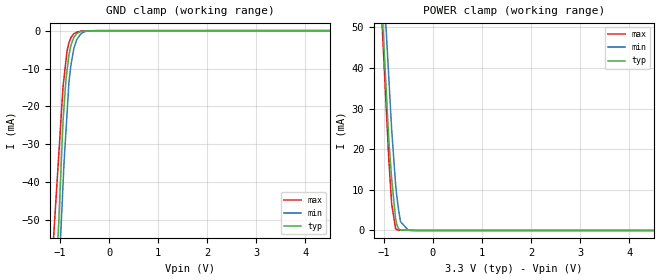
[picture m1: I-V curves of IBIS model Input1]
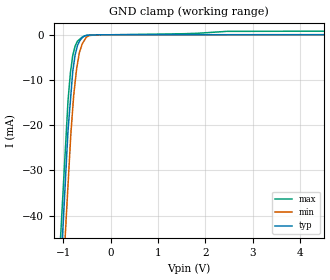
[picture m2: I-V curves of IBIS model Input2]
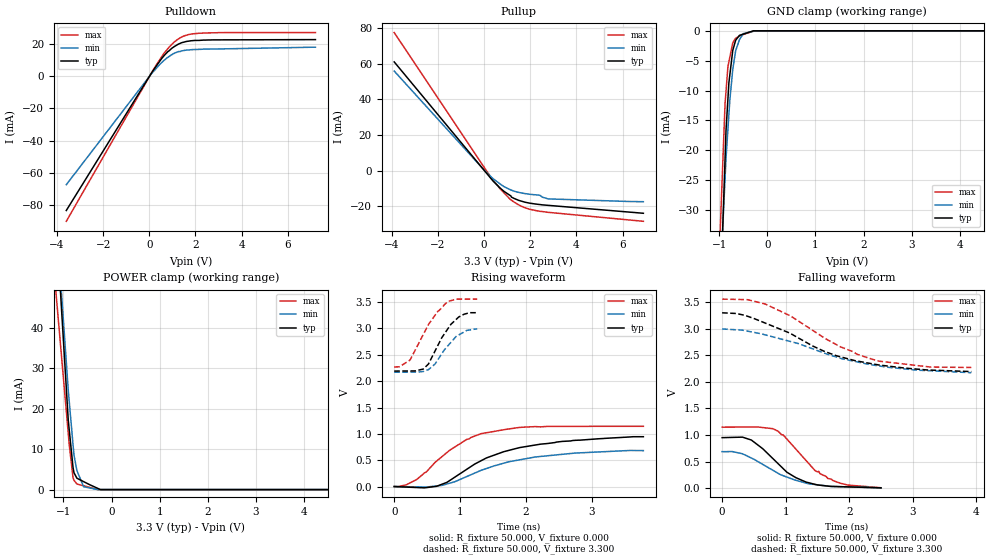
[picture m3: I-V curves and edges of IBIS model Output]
[IBIS Ver]   3.2
[Comment Char] |_char
[File Name]   ads1602ipfbt.ibs
[File Rev]   3.0
[Source]
| This model file was created by Teraspeed Consulting Group LLC
| (http://www.teraspeed.com/).
[Date]   08-30-2006
[Notes]   Quality Check of this IBIS model: Model Passes IBIS Check
   Model parses into ICX IS. Simulation done with Hyperlynx.
   1. MIN TYP MAX information is based on Temprature and Voltage
   characteristics only.
[Disclaimer]
| This model is designed as an aid for customers of Texas Instruments.
| TI and its licensors and suppliers make no warranties, either expressed
| or implied, with respect to this  model, including the warranties of
| merchantability or fitness for a particular purpose.
| The model is provided solely on an "as is" basis. The entire risk as to
| its quality and performance is with the customer.
[Copyright]
| (C) Copyright 2008 Texas Instruments Incorporated. All rights reserved.
[Component] ADS1602IPFBT
[Manufacturer] TI
[Package]
| variable   typ   min   max
R_pkg  1.8006E-02  1.8006E-02  1.8006E-02
L_pkg  2.1607E-09  2.1607E-09  2.1607E-09
C_pkg  6.0021E-13  6.0021E-13  6.0021E-13
[Pin] signal_name  model_name  R_pin  L_pin C_pin
1   AGND   GND   1.89E-02   2.26E-09   6.29E-13
2   AVDD   POWER   1.80E-02   2.16E-09   6.01E-13
3   AGND   GND   1.72E-02   2.06E-09   5.73E-13
4   AINN   Term1   1.64E-02   1.97E-09   5.47E-13
5   AINP   Term1   1.56E-02   1.87E-09   5.21E-13
6   AGND   GND   1.49E-02   1.78E-09   4.96E-13
7   AVDD   POWER   1.49E-02   1.78E-09   4.96E-13
8   RBIAS   Term1   1.56E-02   1.87E-09   5.21E-13
9   AGND   GND   1.64E-02   1.97E-09   5.47E-13
10   AVDD   POWER   1.72E-02   2.06E-09   5.73E-13
11   AGND   GND   1.80E-02   2.16E-09   6.01E-13
12   AVDD   POWER   1.89E-02   2.26E-09   6.29E-13
13   _REFEN  Input2  1.89E-02   2.26E-09   6.29E-13
14   NC   NC   1.80E-02   2.16E-09   6.01E-13
15   RPULLUP Term1   1.72E-02   2.06E-09   5.73E-13
16   NC   NC   1.64E-02   1.97E-09   5.47E-13
17   _PD   Input2  1.56E-02   1.87E-09   5.21E-13
18   DVDD   POWER   1.49E-02   1.78E-09   4.96E-13
19   DGND   GND   1.49E-02   1.78E-09   4.96E-13
20   SYNC   Input2  1.56E-02   1.87E-09   5.21E-13
21   OTR   Output  1.64E-02   1.97E-09   5.47E-13
22   DGND   GND   1.72E-02   2.06E-09   5.73E-13
23   DVDD   POWER   1.80E-02   2.16E-09   6.01E-13
24   NC   NC   1.89E-02   2.26E-09   6.29E-13
25   NC   NC   1.89E-02   2.26E-09   6.29E-13
26   NC   NC   1.80E-02   2.16E-09   6.01E-13
27   _SCLK   Output  1.72E-02   2.06E-09   5.73E-13
28   SCLK   Output  1.64E-02   1.97E-09   5.47E-13
29   _DOUT   Output  1.56E-02   1.87E-09   5.21E-13
30   DOUT   Output  1.49E-02   1.78E-09   4.96E-13
31   _FSO   Output  1.49E-02   1.78E-09   4.96E-13
32   FSO   Output  1.56E-02   1.87E-09   5.21E-13
33   DGND   GND   1.64E-02   1.97E-09   5.47E-13
34   DVDD   POWER   1.72E-02   2.06E-09   5.73E-13
35   NC   NC   1.80E-02   2.16E-09   6.01E-13
36   DGND   GND   1.89E-02   2.26E-09   6.29E-13
37   IOVDD   POWER   1.89E-02   2.26E-09   6.29E-13
38   DGND   GND   1.80E-02   2.16E-09   6.01E-13
39   AGND   GND   1.72E-02   2.06E-09   5.73E-13
40   CLK   Input1  1.64E-02   1.97E-09   5.47E-13
41   AGND   GND   1.56E-02   1.87E-09   5.21E-13
42   AVDD   POWER   1.49E-02   1.78E-09   4.96E-13
43   VCAP   Term1   1.49E-02   1.78E-09   4.96E-13
44   VREFN   Term1   1.56E-02   1.87E-09   5.21E-13
45   VREFN   Term1   1.64E-02   1.97E-09   5.47E-13
46   VMID   Term1   1.72E-02   2.06E-09   5.73E-13
47   VREFP   Term1   1.80E-02   2.16E-09   6.01E-13
48   VREFP   Term1   1.89E-02   2.26E-09   6.29E-13
[Diff Pin] inv_pin vdiff tdelay_typ tdelay_min tdelay_max
5   4   NA  NA  NA  NA
28  27  NA  NA  NA  NA
30  29  NA  NA  NA  NA
32  31  NA  NA  NA  NA
| Models and submodels in the file (4): Input1 (Input), Input2 (Input), Output (Output), Term1 (Terminator)
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[Model] Input1
Model_type Input
Vinl = 990.000mV
Vinh = 2.31000V
C_comp 2.00000pF 2.00000pF 2.00000pF
| variable typ   min   max
[Voltage Range] 3.30000V 3.00000V 3.60000V
[POWER Clamp Reference] 3.30000V 3.00000V 3.60000V
[GND Clamp Reference] 0.00000V 0.00000V 0.00000V
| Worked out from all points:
|   GND clamp passes 1 mA (typ) near -0.67 V on its own axis
|   POWER clamp passes 1 mA (typ) near -0.72 V on its own axis
[GND Clamp]
-3.3V     -742.8mA   -704.3mA   -501mA
-940mV    -23.81mA   -40.58mA   -14.84mA
-920mV    -20.15mA   -34.95mA   -12.5mA
-880mV    -12.82mA   -26.45mA   -7.834mA
-860mV    -10.7mA    -22.2mA    -5.498mA
-820mV    -6.461mA   -13.7mA    -3.17mA
-780mV    -3.9mA     -9.185mA   -1.829mA
-720mV    -1.771mA   -4.71mA    -825.5uA
-660mV    -787.2uA   -2.326mA   -383.3uA
-540mV    -168.5uA   -505.8uA   -71.65uA
-240mV    -9.723uA   -9.634uA   -1.75uA
6.6V      11.72uA    18.06uA    6.055uA
[POWER Clamp]
-3.3V     585.2mA    563.6mA    629.9mA
-1.06V    59.95mA    72.93mA    57.25mA
-1.02V    50.57mA    64.16mA    47.03mA
-900mV    22.43mA    37.88mA    17.72mA
-840mV    12.66mA    24.74mA    6.473mA
-760mV    2.906mA    11.27mA    428uA
-740mV    1.575mA    8.921mA    253.9uA
-700mV    404.3uA    5.099mA    76.65uA
-660mV    92.03uA    2.156mA    70.39uA
-500mV    47.41uA    57.43uA    45.36uA
6.6V      0A         0A         0A
[Model] Input2
Model_type Input
Vinl = 990.000mV
Vinh = 2.31000V
C_comp 2.00000pF 2.00000pF 2.00000pF
| variable typ   min   max
[Voltage Range] 3.30000V 3.00000V 3.60000V
[POWER Clamp Reference] 3.30000V 3.00000V 3.60000V
[GND Clamp Reference] 0.00000V 0.00000V 0.00000V
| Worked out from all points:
|   GND clamp passes 1 mA (typ) near -0.63 V on its own axis
[GND Clamp]
|  Voltage   I(typ)   I(min)   I(max)
-3.3V     -503.8mA   -490.3mA   -476.1mA
-900mV    -21.11mA   -33.25mA   -14.54mA
-840mV    -13.29mA   -21.82mA   -7.65mA
-800mV    -8.085mA   -16.2mA    -4.572mA
-780mV    -6.626mA   -13.39mA   -3.734mA
-750mV    -4.437mA   -10.5mA    -2.477mA
-720mV    -3.188mA   -7.613mA   -1.838mA
-660mV    -1.507mA   -3.925mA   -1.049mA
-550mV    -282.4uA   -1.149mA   -273.1uA
-440mV    -79.83uA   -142.4uA   -129uA
-220mV    -6.361uA   -5.894uA   -40uA
6.6V      14.04uA    12.24uA    839.7uA
[POWER Clamp]
-3.3V     0A         0A         0A
6.6V      0A         0A         0A
[Model] Output
Model_type Output
Vref=0.00000V
Rref=5.00000Mohms
Cref=0.00000F
Vmeas=1.65000V
C_comp 2.00000pF 2.00000pF 2.00000pF
| variable typ   min   max
[Voltage Range] 3.30000V 3.00000V 3.60000V
[POWER Clamp Reference] 3.30000V 3.00000V 3.60000V
[Pullup Reference] 3.30000V 3.00000V 3.60000V
[Pulldown Reference] 0.00000V 0.00000V 0.00000V
[GND Clamp Reference] 0.00000V 0.00000V 0.00000V
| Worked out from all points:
|   slope of the pulldown table from 0 to 0.495 V, typ, clamps not added: 47.7 ohm
|   slope of the pullup table from 0 to 0.495 V, typ, clamps not added: 66.9 ohm
|   GND clamp passes 1 mA (typ) near -0.60 V on its own axis
|   POWER clamp passes 1 mA (typ) near -0.41 V on its own axis
|   rising waveform, R_fixture 50.000, V_fixture 0.000: 20-80 % time 1.05ns typ, 1.07ns min, 714ps max; typ from 0.006 V to 0.95 V
|   falling waveform, R_fixture 50.000, V_fixture 0.000: 20-80 % time 548ps typ, 690ps min, 585ps max; typ from 0.95 V to 0.006 V
|   falling waveform, R_fixture 50.000, V_fixture 3.300: 20-80 % time 1.31ns typ, 1.43ns min, 1.14ns max; typ from 3.3 V to 2.19 V
|   rising waveform, R_fixture 50.000, V_fixture 3.300: 20-80 % time 304ps typ, 301ps min, 355ps max; typ from 2.19 V to 3.3 V
[GND Clamp]
-3.6V     -671.8mA   -487.7mA   -586.5mA
-3V       -528.4mA   -385.6mA   -459.8mA
-880mV    -21.47mA   -24.75mA   -12.22mA
-860mV    -16.69mA   -21.34mA   -10.14mA
-820mV    -11.37mA   -16.46mA   -5.974mA
-800mV    -8.704mA   -14.02mA   -5.185mA
-780mV    -7.354mA   -11.57mA   -4.396mA
-720mV    -3.302mA   -6.494mA   -2.028mA
-660mV    -1.589mA   -3.363mA   -1.234mA
-500mV    -548.3uA   -478.1uA   -619.2uA
-270mV    0A         -38.25uA   0A
7.2V      0A         0A         0A
[Pulldown]
-3.6V     -83.44mA   -67.43mA   -90.14mA
140mV     2.973mA    2.239mA    3.125mA
640mV     12.72mA    9.781mA    14.21mA
980mV     17.33mA    13.34mA    19.74mA
1.22V     19.5mA     15.01mA    22.68mA
1.44V     20.86mA    15.73mA    24.53mA
1.72V     21.72mA    16.18mA    25.83mA
2.36V     22.34mA    16.72mA    26.75mA
7.2V      22.63mA    17.95mA    27.01mA
[Pullup]
|  Voltage   I(typ)   I(min)   I(max)
-3.9V     60.97mA    55.83mA    77.43mA
0V        97.14uA    239.5uA    1.807mA
300mV     -4.585mA   -3.553mA   -3.954mA
720mV     -10.18mA   -7.819mA   -10.71mA
1.16V     -14.31mA   -10.92mA   -16.51mA
1.18V     -14.89mA   -11.01mA   -16.68mA
1.3V      -15.68mA   -11.59mA   -17.72mA
1.76V     -17.74mA   -12.93mA   -20.86mA
2.4V      -19.07mA   -13.83mA   -22.86mA
2.54V     -19.29mA   -15.03mA   -23.05mA
2.78V     -19.55mA   -15.93mA   -23.47mA
6.9V      -23.98mA   -17.49mA   -28.49mA
[POWER Clamp]
-3.9V     606.6mA    538.6mA    422.6mA
-1.14V    64.33mA    65.7mA     46.6mA
-1.06V    48.61mA    52mA       35.71mA
-970mV    30.93mA    36.58mA    23.44mA
-900mV    17.18mA    24.58mA    13.91mA
-880mV    14.82mA    21.87mA    11.18mA
-800mV    5.406mA    11.01mA    2.89mA
-780mV    4.158mA    8.472mA    2.298mA
-720mV    2.815mA    4.701mA    1.381mA
-580mV    1.97mA     710.8uA    976.2uA
-230mV    0A         0A         0A
6.9V      0A         0A         0A
[Rising Waveform]
R_fixture = 50.000
V_fixture = 0.000
V_fixture_min = 0.000
V_fixture_max = 0.000
|  time   V(typ)   V(min)   V(max)
0s        6.072mV    6.82mV     8.158mV
180ps     -3.481mV   3.037mV    36.74mV
340ps     -11.97mV   -326.8uV   138.7mV
640ps     10.32mV    16.91mV    484.3mV
800ps     85.89mV    55.34mV    650.4mV
1.1ns     332.4mV    195.3mV    898.3mV
1.32ns    496.3mV    314.4mV    1.008V
1.66ns    665.5mV    448mV      1.081V
2.22ns    809mV      575.9mV    1.136V
3.78ns    949.7mV    686.6mV    1.147V
[Falling Waveform]
R_fixture = 50.000
V_fixture = 0.000
V_fixture_min = 0.000
V_fixture_max = 0.000
|  time   V(typ)   V(min)   V(max)
0s        949.7mV    686.6mV    1.147V
320ps     959.7mV    647.1mV    1.149V
460ps     905mV      566.8mV    1.15V
800ps     555mV      335.9mV    1.118V
1.02ns    299mV      208.4mV    922.1mV
1.32ns    114.9mV    95.77mV    520.9mV
1.46ns    72.61mV    68.56mV    333.6mV
1.66ns    39.55mV    40.59mV    183.8mV
1.86ns    28.66mV    27.64mV    92.84mV
2.5ns     6.072mV    6.82mV     8.158mV
[Falling Waveform]
R_fixture = 50.000
V_fixture = 3.300
V_fixture_min = 3.000
V_fixture_max = 3.600
|  time   V(typ)   V(min)   V(max)
0s        3.297V     2.993V     3.554V
360ps     3.249V     2.961V     3.545V
680ps     3.103V     2.882V     3.461V
1.08ns    2.905V     2.756V     3.235V
1.6ns     2.576V     2.542V     2.83V
2.12ns    2.391V     2.375V     2.519V
2.36ns    2.339V     2.317V     2.424V
2.48ns    2.314V     2.296V     2.386V
3.28ns    2.22V      2.207V     2.277V
3.92ns    2.192V     2.171V     2.269V
[Rising Waveform]
R_fixture = 50.000
V_fixture = 3.300
V_fixture_min = 3.000
V_fixture_max = 3.600
|  time   V(typ)   V(min)   V(max)
0s        2.192V     2.171V     2.269V
80ps      2.193V     2.171V     2.274V
240ps     2.194V     2.172V     2.4V
440ps     2.23V      2.184V     2.882V
520ps     2.326V     2.22V      3.075V
620ps     2.573V     2.326V     3.25V
820ps     3.004V     2.678V     3.515V
980ps     3.217V     2.877V     3.554V
1.1ns     3.282V     2.962V     3.554V
1.26ns    3.297V     2.993V     3.554V
[Ramp]
| variable typ min max
dV/dt_r 566.165m/1.00211n 407.853m/1.12868n 684.243m/797.688p
dV/dt_f 663.371m/1.30000n 493.365m/1.41583n 771.381m/1.14731n
R_load = 50.0000Ohms
